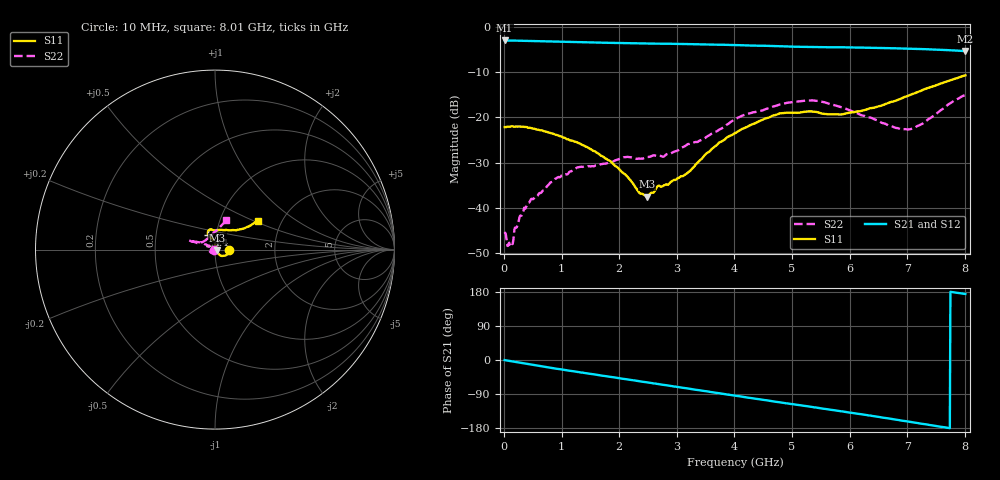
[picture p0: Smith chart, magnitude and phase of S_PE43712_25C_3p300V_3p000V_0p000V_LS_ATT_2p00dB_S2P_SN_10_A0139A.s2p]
! DEVICE ID: PE43712
! File Path: z:\PE43713\PE43713_CHAR_NOM_04292014\AMB\3p300\LS_ATT_2p00dB\PE43713_AMB_3p300V_3p000V_0p000V_LS_ATT_2p00dB_S2P_SN_10_A0139A.s2p
! Serial: 10
! Lot: A0139A
! Temp: 25C
! VDD: 3.300
! VSS: 0.000
! Control_Hi: 3.000
! Control_Lo: 0.000
! Attenuation Step: 2.00dB
! Port 1: RF1
! Port 2: RF2
! ThroughPath:1-2
! IDD: 0.0001466933
! ISS: -9.96e-008
#  Hz  S  RI  R  50
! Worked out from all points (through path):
!   801 points, 10 MHz to 8.01 GHz, reference 50 ohm
!   highest |S21| = -3.02 dB at 10 MHz (marker M1); lowest = -5.4 dB at 8.01 GHz (marker M2)
!   group delay of S21, straight-line fit = 63.6 ps
!   lowest |S11| = -37.5 dB at 2.48 GHz (marker M3), VSWR 1.03, Z = 51.3 - j0.19 ohm
!   |S11| at or under -10 dB: start of sweep to end of sweep
!   |S22| runs from -48.5 to -15.1 dB; largest |S21 - S12| = 0.002
!   S11 on the Smith chart (normalised r, x): 10 MHz: 1.17, -0.00; 4.4 GHz: 0.92, +0.15; 8.01 GHz: 1.52, +0.54
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1e7  0.078 -0.000427  0.7064 -0.00394  0.7061 -0.00383  -0.00517 -0.000184
1.1e8  0.0788 -0.00453  0.7039 -0.0367  0.7036 -0.0366  -0.00361 -0.00105
2.9e8  0.0771 -0.0162  0.6951 -0.0939  0.6945 -0.094  -0.00403 -0.00713
4.4e8  0.0731 -0.0222  0.6841 -0.1395  0.6833 -0.1393  -0.00454 -0.0106
9e8  0.0545 -0.0334  0.6322 -0.2647  0.6321 -0.2645  -0.0138 -0.0158
1.35e9  0.0357 -0.0347  0.5645 -0.3686  0.5643 -0.3686  -0.0232 -0.0163
1.85e9  0.0212 -0.0247  0.4738 -0.4664  0.4737 -0.4662  -0.0308 -0.00804
2.1e9  0.0145 -0.0184  0.4223 -0.5084  0.4224 -0.5082  -0.0361 -0.00327
2.35e9  0.0126 -0.00734  0.3669 -0.5449  0.367 -0.5448  -0.0348 0.00395
2.48e9  0.0132 -0.00185  0.3368 -0.5609  0.3368 -0.5609  -0.0347 0.0105
2.68e9  0.0149 0.00923  0.291 -0.5818  0.2911 -0.5817  -0.0309 0.0217
3.15e9  0.00421 0.023  0.1739 -0.6208  0.1741 -0.6207  -0.0421 0.0237
3.71e9  -0.00744 0.0499  0.0319 -0.6328  0.0317 -0.633  -0.0627 0.0336
4.01e9  -0.0204 0.0637  -0.0449 -0.6268  -0.0446 -0.6267  -0.0861 0.0405
4.4e9  -0.0375 0.0804  -0.1382 -0.6032  -0.1376 -0.6032  -0.1068 0.0441
4.8e9  -0.0382 0.1039  -0.2286 -0.5655  -0.2281 -0.5657  -0.1308 0.0475
5.35e9  -0.0248 0.1131  -0.334 -0.4949  -0.3338 -0.4944  -0.1452 0.0514
5.85e9  0.00859 0.107  -0.4204 -0.4191  -0.4197 -0.4194  -0.1214 0.0434
6.68e9  0.0958 0.108  -0.5233 -0.2506  -0.5231 -0.2504  -0.0688 0.0423
6.9e9  0.12 0.1083  -0.5409 -0.2004  -0.5406 -0.2003  -0.0512 0.0524
7.1e9  0.1413 0.1135  -0.5519 -0.1529  -0.5513 -0.1529  -0.0327 0.0682
8.01e9  0.2415 0.1621  -0.5363 0.0544  -0.5347 0.0534  0.0628 0.165
